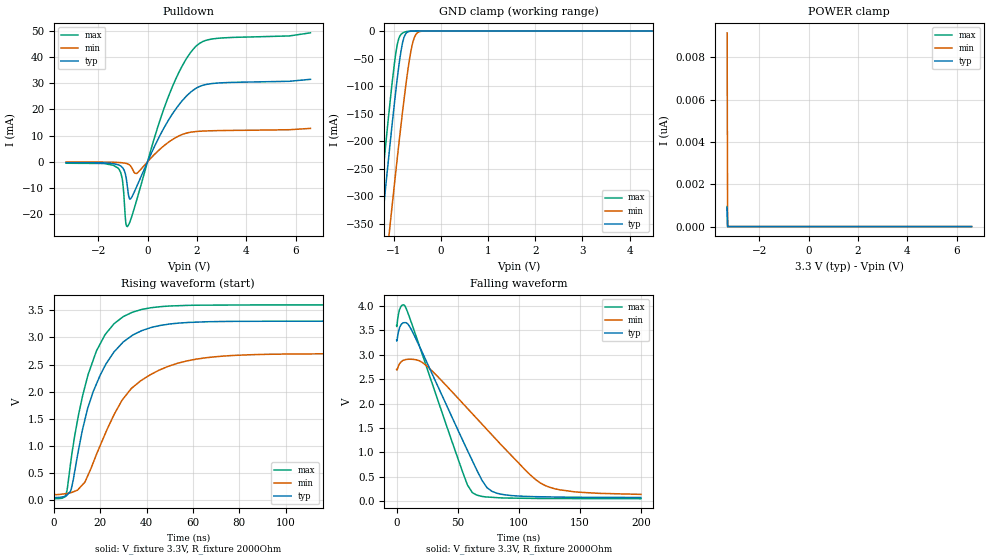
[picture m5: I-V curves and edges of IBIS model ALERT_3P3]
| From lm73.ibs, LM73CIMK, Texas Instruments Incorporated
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|   (nom PVT)   (slow PVT)   (fast PVT)
|   Model ALERT_3P3
[Model]   ALERT_3P3
Model_type   Open_drain
Polarity   Non-Inverting
Vmeas = 1.65
Vref = 3.3
Cref = 1pF
Rref = 2000
|   typ   min   max
|   (nom PVT)   (fast PVT)   (slow PVT)
C_comp   0.708p   0.656p   0.778p
|C_comp (ON state)   0.791p   0.790p   0.808p
|C_comp (OFF state)   0.708p   0.656p   0.778p
[Voltage Range]   3.3   2.7   3.6
[Temperature Range]   27   150   -40
[Pullup Reference]   3.3   2.7   3.6
[Pulldown Reference]   0   0   0
[Power Clamp Reference]   3.3   2.7   3.6
[GND Clamp Reference]   0   0   0
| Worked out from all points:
|   slope of the pulldown table from 0 to 0.495 V, typ, clamps not added: 50 ohm
|   GND clamp passes 1 mA (typ) near -0.68 V on its own axis
|   falling waveform, V_fixture 3.3V, R_fixture 2000Ohm: 20-80 % time 35.8ns typ, 57.4ns min, 29.1ns max; typ from 3.3 V to 0.075 V
|   rising waveform, V_fixture 3.3V, R_fixture 2000Ohm: 20-80 % time 14.9ns typ, 20.5ns min, 12.6ns max; typ from 0.074 V to 3.3 V
[Pulldown]
|   Voltage   I(typ)   I(min)   I(max)
-3.3V     -353.1uA   -104.8uA   -552uA
-1.191V   -1.131mA   -257.4uA   -2.419mA
-1.023V   -2.109mA   -377.9uA   -6.557mA
-884.4mV  -5.173mA   -584.2uA   -22.88mA
-815.1mV  -9.547mA   -777uA     -24.77mA
-676.5mV  -14.09mA   -1.717mA   -22.01mA
-429mV    -9.265mA   -4.433mA   -14.32mA
848.1mV   15.89mA    7.459mA    24.97mA
1.403V    23.3mA     10.41mA    36.57mA
1.957V    28.05mA    11.55mA    44.1mA
2.788V    30.05mA    11.9mA     47.14mA
6.6V      31.52mA    12.76mA    49.29mA
[GND Clamp]
|   Voltage   I(typ)   I(min)   I(max)
-3.3V     -2.187A    -2.243A    -2.165A
-1.379V   -462.3mA   -601.4mA   -389.9mA
-1.29V    -384.4mA   -526.6mA   -310.1mA
-1.201V   -307.5mA   -452.4mA   -231.7mA
-1.112V   -232.1mA   -379.1mA   -155.6mA
-1.053V   -183.2mA   -330.8mA   -107.4mA
-924mV    -84.31mA   -228.8mA   -23.73mA
-844.8mV  -35.09mA   -168.7mA   -5.855mA
-785.4mV  -12.04mA   -125.8mA   -2.445mA
-607.2mV  -150.1uA   -24.34mA   -45.96uA
-438.9mV  -1.21uA    -737.9uA   -131.7nA
6.6V      0A         0A         0A
[POWER Clamp]
|   Voltage   I(typ)   I(min)   I(max)
-3.3V     912.3pA    9.166nA    952.2pA
-3.28V    0A         0A         0A
-3.27V    0A         0A         0A
6.6V      0A         0A         0A
[Ramp]
R_load = 2000
|   typ   min   max
dV/dt_r   1.93581/1.4945e-08   1.54562/2.04709e-08   2.12962/1.26e-08
dV/dt_f   1.93486/3.57959e-08   1.53628/5.74136e-08   2.12935/2.91039e-08
[Falling Waveform]
V_fixture = 3.3V
V_fixture_min = 2.7V
V_fixture_max = 3.6V
R_fixture = 2000Ohm
C_fixture = 0F
|   Time   V(typ)   V(min)   V(max)
0s        3.3V       2.7V       3.6V
3.507ns   3.61V      2.851V     3.992V
7.862ns   3.656V     2.905V     3.949V
22.89ns   2.947V     2.81V      2.871V
53.96ns   1.254V     2.01V      601.6mV
61.96ns   829.8mV    1.793V     175mV
69.97ns   422.1mV    1.576V     97.8mV
77.97ns   202.6mV    1.359V     79.15mV
121.4ns   89.18mV    321.7mV    55.11mV
199.9ns   75.23mV    139.5mV    51.08mV
[Rising Waveform]
V_fixture = 3.3V
V_fixture_min = 2.7V
V_fixture_max = 3.6V
R_fixture = 2000Ohm
C_fixture = 0F
|   Time   V(typ)   V(min)   V(max)
0s        73.64mV    123.9mV    50.62mV
4.826ns   70.39mV    116.7mV    59.59mV
7.52ns    202.8mV    139.2mV    769.7mV
12.48ns   1.319V     288.3mV    1.938V
18.36ns   2.14V      839.9mV    2.75V
25.96ns   2.734V     1.576V     3.254V
33.96ns   3.042V     2.078V     3.467V
49.42ns   3.244V     2.469V     3.578V
69.42ns   3.292V     2.643V     3.596V
199.9ns   3.3V       2.7V       3.6V
